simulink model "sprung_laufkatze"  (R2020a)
settings: Solver=ode45  StartTime=0.0  StopTime=20  RelTol=1e-3  EnableMultiTasking=on

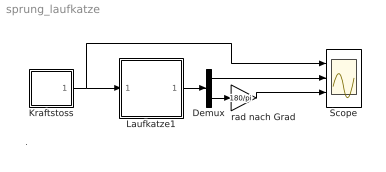
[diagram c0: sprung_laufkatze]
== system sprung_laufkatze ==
  note: .
  Demux : Demux  Outputs=2
  Kraftstoss : Subsystem  mask(Kraftstoss){tS=1, dt=10, Fmax=1}
      mask prompts: tS "Startzeit"; dt "Dauer"; Fmax "Staerke"
      mask help: Gibt einen Kraftstoss in Form eines Rechteckimpulses aus.
  Laufkatze1 : Subsystem  mask(Laufkatze){mk=100, ml=10, l=1, g=9.81}
      mask prompts: mk "Laufkatzenmasse"; ml "Lastmasse"; l "Seillaenge"; g "Erdbeschleunigung"
      mask help: Modell einer Laufkatze als Regelstrecke
  Scope : Scope  NumInputPorts=3
  rad nach Grad : Gain  Gain=180/pi
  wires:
  Kraftstoss/1(Fext) -> Scope/1, Laufkatze1/1(u)
  Laufkatze1/1(x,th) -> Demux/1
  Demux/2 -> rad nach Grad/1
  rad nach Grad/1 -> Scope/3
  Demux/1 -> Scope/2

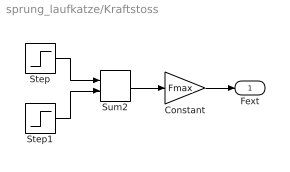
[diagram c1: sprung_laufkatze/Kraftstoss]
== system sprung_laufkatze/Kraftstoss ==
  Constant : Gain  Gain=Fmax  SaturateOnIntegerOverflow=on
  Step : Step  Time=tS  SampleTime=0
  Step1 : Step  Time=tS+dt  After=-1  SampleTime=0
  Sum2 : Sum  InputSameDT=on  SaturateOnIntegerOverflow=on
  Fext : Outport
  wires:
  Constant/1 -> Fext/1
  Step1/1 -> Sum2/2
  Step/1 -> Sum2/1
  Sum2/1 -> Constant/1

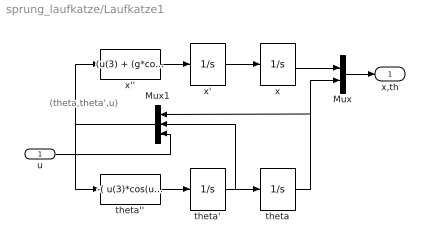
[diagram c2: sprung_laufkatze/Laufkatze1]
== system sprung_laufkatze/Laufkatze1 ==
  note: (theta,theta',u)
  u : Inport
  Mux : Mux  Inputs=2
  Mux1 : Mux  Inputs=3
  theta : Integrator
  theta' : Integrator
  theta'' : Fcn  Expr=-( u(3)*cos(u(1)) + (g + l*u(2)^2*cos(u(1)))*ml*sin(u(1)) + g*mk*sin(u(1)) ) / ( (mk + ml*sin(u(1))^2)*l )
  x : Integrator
  x' : Integrator
  x'' : Fcn  Expr=(u(3) + (g*cos(u(1)) + l*u(2)^2)*ml*sin(u(1)))/(mk + ml*sin(u(1))^2)
  x,th : Outport
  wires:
  theta''/1 -> theta'/1
  x''/1 -> x'/1
  u/1 -> Mux1/3
  theta'/1 -> Mux1/2, theta/1
  x'/1 -> x/1
  Mux1/1 -> theta''/1, x''/1
  theta/1 -> Mux1/1, Mux/2
  x/1 -> Mux/1
  Mux/1 -> x,th/1
